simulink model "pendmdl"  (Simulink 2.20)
settings: Solver=ode45  StartTime=0.0  StopTime=4.0  RelTol=1e-6  AbsTol=1e-6
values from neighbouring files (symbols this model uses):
  alpha = m*L/(J+m*L^2)    (= 2)    [PENDOL2.M]    (also in PENDOLO.M)
  g = 9.81    [PENDOL2.M]    (also in PENDOLO.M)
  K = M*[alpha*g+lam1*lam2 -(lam1+lam2)]/alpha    [PENDOL2.M]    (also in PENDOLO.M)
  M = 2    [PENDOL2.M]    (also in PENDOLO.M)
  thdot0 = th00    (= 0.1)    [PENDOL2.M]    (also in PENDOLO.M = 1)
undefined symbols (not defined in the file or in its folder): th0
libraries: simulink x1

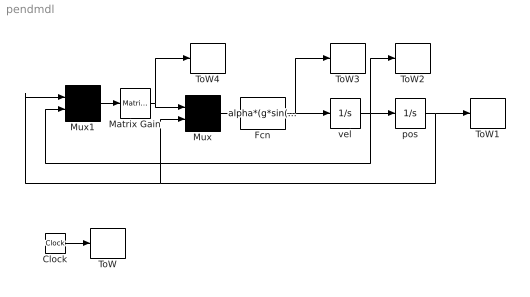
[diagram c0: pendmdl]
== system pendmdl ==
  Clock : Clock
  Fcn : Fcn  Expr=alpha*(g*sin(u(2))-u(1)*cos(u(2))/M)
  Matrix Gain : simulink/Linear/Matrix Gain  K=K
  Mux : Mux  Inputs=2
  Mux1 : Mux  Inputs=2
  ToW : ToWorkspace  VariableName=t  SampleTime=-1
  ToW1 : ToWorkspace  VariableName=th  SampleTime=-1
  ToW2 : ToWorkspace  VariableName=thdot  SampleTime=-1
  ToW3 : ToWorkspace  VariableName=thddot  SampleTime=-1
  ToW4 : ToWorkspace  VariableName=u  SampleTime=-1
  pos : Integrator  ExternalReset=none  InitialConditionSource=internal  InitialCondition=th0  LimitOutput=off  UpperSaturationLimit=inf  LowerSaturationLimit=-inf  ShowSaturationPort=off  ShowStatePort=off  AbsoluteTolerance=auto
  vel : Integrator  ExternalReset=none  InitialConditionSource=internal  InitialCondition=thdot0  LimitOutput=off  UpperSaturationLimit=inf  LowerSaturationLimit=-inf  ShowSaturationPort=off  ShowStatePort=off  AbsoluteTolerance=auto
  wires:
  Mux/1 -> Fcn/1
  vel/1 -> pos/1, ToW2/1, Mux1/2
  Fcn/1 -> vel/1, ToW3/1
  Clock/1 -> ToW/1
  Mux1/1 -> Matrix Gain/1
  pos/1 -> ToW1/1, Mux1/1, Mux/2
  Matrix Gain/1 -> Mux/1, ToW4/1
